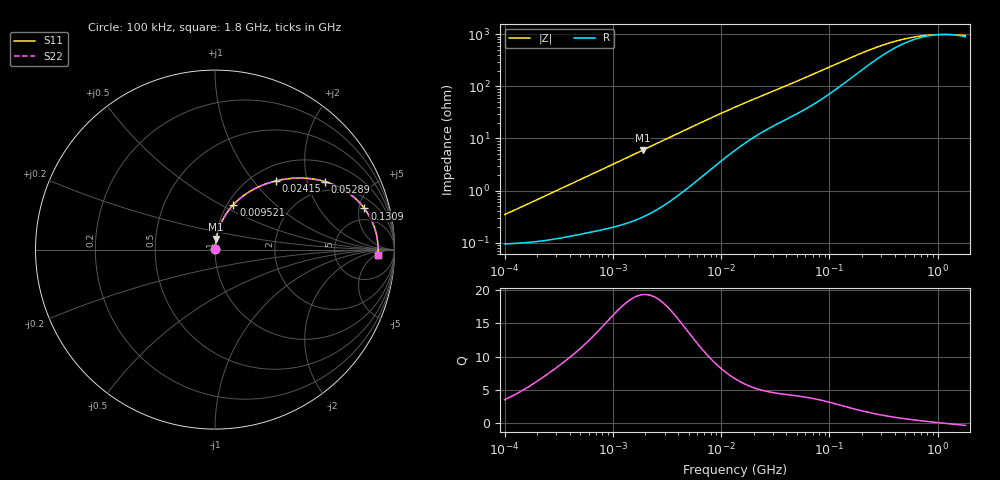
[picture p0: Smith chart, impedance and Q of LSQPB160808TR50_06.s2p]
! LSQPB160808TR50_06  S-PARAMETER MODEL  ( General Type )
! Model Generated by TAIYO YUDEN Corporation (http://www.ty-top.com)
! Version 1.0
! TAIYO YUDEN Control No. 110726NG25SE-FKC
! Copyright(c) 2011 TAIYO YUDEN CO.,LTD. All Rights Reserved.
! Product Description (link to TY-COMPAS)
! https://ds.yuden.co.jp/TYCOMPAS/or/detail?pn=LSQPB160808TR50M06&u=M
! Products Name : Inductors
! Characteristics :
!  Inductance : 0.50 uH , SRF(min) : 710 MHz , DC Resistance(max) : 0.117 Ohm
!  Rated Current : Saturation :1200 mA , Temp Rise : 1050 mA (40 degC)
!  Case Size : 1.6 x 0.8 / 0.063 x 0.031 [mm/inch] , Thickness : 0.8 / 0.031 [mm/inch]
!  (Conditions: Temperature = 25 degC , DC Bias Current/Voltage = 0A / 0V)
! External Node Assignments :
!  1  o---GGG---o  2
! GND o---------o GND
! Frequency Range : 0.1MHz  -  1800MHz  [ 402 STEP ]
# MHz S RI R 50
! Freq[MHz].  S11 Real  S11 Imag  S21 Real  S21 Imag  S12 Real  S12 Imag  S22 Real  S22 Imag
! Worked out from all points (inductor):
!   401 points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, 100 kHz to 1.8 GHz, reference 50 ohm
!   read as one part in series: L = 528 nH near 105 kHz
!   highest Q = 19.3 at 1.891 MHz (marker M1), where L = 503 nH
!   self-resonance near 1.147 GHz
!   S11 on the Smith chart (normalised r, x): 100 kHz: 1.00, +0.01; 9.521 MHz: 1.07, +0.58; 24.15 MHz: 1.27, +1.32; 52.89 MHz: 1.64, +2.57; 130.9 MHz: 3.16, +5.68; 1.8 GHz: 19, -6
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0.1  0.000952 0.00332  0.999 -0.00332  0.999 -0.00332  0.000952 0.00332
0.134171  0.000991 0.00444  0.999 -0.00444  0.999 -0.00444  0.000991 0.00444
0.516129  0.00173 0.0166  0.9983 -0.0166  0.9983 -0.0166  0.00173 0.0166
1.050184  0.00312 0.0332  0.9969 -0.0332  0.9969 -0.0332  0.00312 0.0332
1.890522  0.0066 0.0591  0.9934 -0.0591  0.9934 -0.0591  0.0066 0.0591
2.66389  0.0114 0.0825  0.9886 -0.0825  0.9886 -0.0825  0.0114 0.0825
5.554714  0.0413 0.1634  0.9587 -0.1634  0.9587 -0.1634  0.0413 0.1634
9.52142  0.103 0.2508  0.897 -0.2508  0.897 -0.2508  0.103 0.2508
13.41641  0.1716 0.3095  0.8284 -0.3095  0.8284 -0.3095  0.1716 0.3095
17.56533  0.2421 0.3493  0.7579 -0.3493  0.7579 -0.3493  0.2421 0.3493
24.15197  0.3402 0.3829  0.6598 -0.3829  0.6598 -0.3829  0.3402 0.3829
36.62703  0.4832 0.3985  0.5168 -0.3985  0.5168 -0.3985  0.4832 0.3985
52.8901  0.6116 0.3793  0.3884 -0.3793  0.3884 -0.3793  0.6116 0.3793
69.24595  0.6965 0.345  0.3035 -0.345  0.3035 -0.345  0.6965 0.345
95.21179  0.7768 0.2895  0.2232 -0.2895  0.2232 -0.2895  0.7768 0.2895
130.9143  0.8322 0.2293  0.1678 -0.2293  0.1678 -0.2293  0.8322 0.2293
203.4578  0.8758 0.1548  0.1242 -0.1548  0.1242 -0.1548  0.8758 0.1548
357.3983  0.8991 0.085  0.1009 -0.085  0.1009 -0.085  0.8991 0.085
542.0029  0.9056 0.0487  0.0944 -0.0487  0.0944 -0.0487  0.9056 0.0487
802.0705  0.9082 0.0217  0.0918 -0.0217  0.0918 -0.0217  0.9082 0.0217
1186.925  0.9089 -0.00203  0.0911 0.00203  0.0911 0.00203  0.9089 -0.00203
1800  0.9082 -0.0277  0.0918 0.0277  0.0918 0.0277  0.9082 -0.0277
